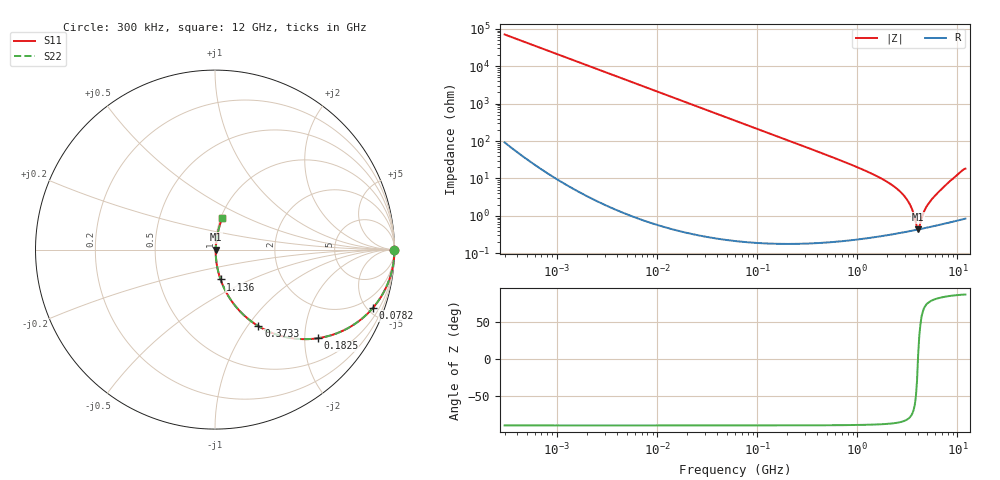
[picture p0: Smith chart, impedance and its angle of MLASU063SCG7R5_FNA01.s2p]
! MLASU063SCG7R5_FNA01  S-PARAMETER MODEL  ( Standard Model )
! Model Generated by TAIYO YUDEN Corporation (http://www.ty-top.com)
! Version 1.0
! TAIYO YUDEN Control No. 240819
! Copyright(c) 2024 TAIYO YUDEN CO.,LTD. All Rights Reserved.
! Product Description (link to TY-COMPAS)
! https://ds.yuden.co.jp/TYCOMPAS/or/detail?pn=MLASU063SCG7R5DFNA01&u=M
! Products Name : Multilayer Ceramic Capacitors
! Characteristics :
!  Capacitance : 7.5 [pF] , Rated Voltage : 50 [V] , TCC : CG / C0G
!  Case Size : 0.6 x 0.3 / 0.024 x 0.012 [mm/inch] , Thickness : 0.3 / 0.012 [mm/inch]
!  (Conditions: Temperature = 25 [degC] , DC Bias Voltage = 0 [V])
! External Node Assignments :
!  1  o---| |---o  2
! GND o---------o GND
! Frequency Range : 0.3MHz  -  12000MHz  [ 401 STEP ]
# MHZ S RI R 50
! Freq[MHz].  S11 Real  S11 Imag  S21 Real  S21 Imag  S12 Real  S12 Imag  S22 Real  S22 Imag
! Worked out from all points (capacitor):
!   401 points, 300 kHz to 12 GHz, reference 50 ohm
!   read as one part in series: C = 7.5 pF near 316.3 kHz
!   lowest |Z| = 434 mohm at 4.05 GHz (marker M1)
!   series resonance near 4.033 GHz, so ESL is about 210 pH
!   S11 on the Smith chart (normalised r, x): 300 kHz: open; 78.2 MHz: 1.00, -5.42; 182.5 MHz: 1.00, -2.32; 373.3 MHz: 1.00, -1.13; 1.136 GHz: 1.00, -0.34; 12 GHz: 1.02, +0.36
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0.3  1 -0.00141  3.83e-06 0.00141  3.83e-06 0.00141  1 -0.00141
1.769972  0.9999 -0.00834  7.24e-05 0.00834  7.24e-05 0.00834  0.9999 -0.00834
10.44266  0.9976 -0.0491  0.00243 0.0491  0.00243 0.0491  0.9976 -0.0491
27.10171  0.9839 -0.1257  0.0161 0.1257  0.0161 0.1257  0.9839 -0.1257
60  0.9258 -0.2619  0.0742 0.2619  0.0742 0.2619  0.9258 -0.2619
78.19928  0.8801 -0.3245  0.1199 0.3245  0.1199 0.3245  0.8801 -0.3245
182.544  0.5734 -0.4938  0.4266 0.4938  0.4266 0.4938  0.5734 -0.4938
353.9943  0.2619 -0.4381  0.7381 0.4381  0.7381 0.4381  0.2619 -0.4381
373.2558  0.2417 -0.4265  0.7583 0.4265  0.7583 0.4265  0.2417 -0.4265
617.4538  0.1026 -0.3005  0.8974 0.3005  0.8974 0.3005  0.1026 -0.3005
1135.593  0.031 -0.1663  0.969 0.1663  0.969 0.1663  0.031 -0.1663
2088.533  0.00854 -0.0735  0.9915 0.0735  0.9915 0.0735  0.00854 -0.0735
2650.866  0.0055 -0.0451  0.9945 0.0451  0.9945 0.0451  0.0055 -0.0451
3107.553  0.0045 -0.0276  0.9955 0.0276  0.9955 0.0276  0.0045 -0.0276
3454.93  0.00421 -0.0163  0.9958 0.0163  0.9958 0.0163  0.00421 -0.0163
3841.137  0.0042 -0.00519  0.9958 0.00519  0.9958 0.00519  0.0042 -0.00519
4050.141  0.00429 0.000468  0.9957 -0.000468  0.9957 -0.000468  0.00429 0.000468
4270.516  0.00444 0.00476  0.9956 -0.00476  0.9956 -0.00476  0.00444 0.00476
4875.354  0.00503 0.0163  0.995 -0.0163  0.995 -0.0163  0.00503 0.0163
5565.855  0.0059 0.0274  0.9941 -0.0274  0.9941 -0.0274  0.0059 0.0274
8281.503  0.013 0.08  0.987 -0.08  0.987 -0.08  0.013 0.08
12000  0.0397 0.1736  0.9603 -0.1736  0.9603 -0.1736  0.0397 0.1736
